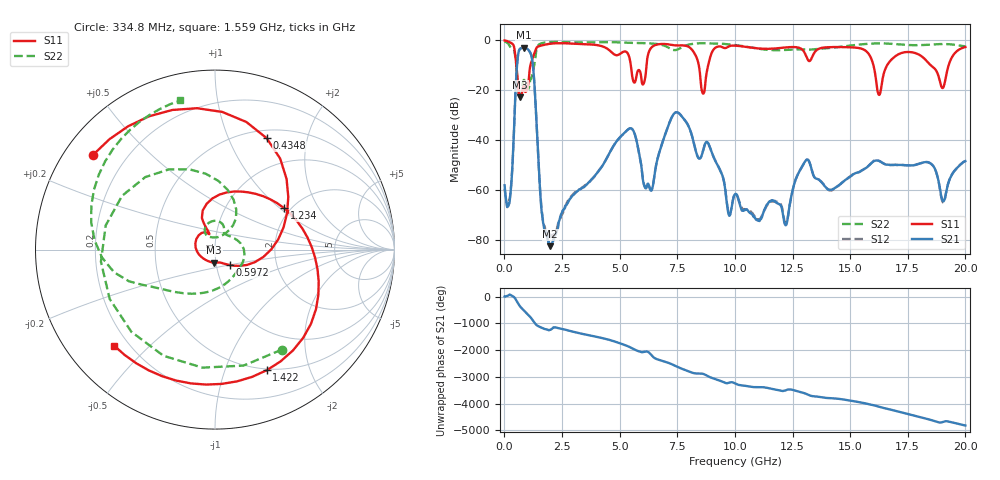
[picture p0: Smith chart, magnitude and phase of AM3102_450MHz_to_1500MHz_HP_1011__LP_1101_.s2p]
!Agilent Technologies,E8364B,MY43040894,A.07.50.67
!Agilent E8364B: A.07.50.67
!Date: Thursday, January 11, 2018 06:26:22
!Correction: S11(Full 2 Port(1,2))
!S21(Full 2 Port(1,2))
!S12(Full 2 Port(1,2))
!S22(Full 2 Port(1,2))
!S2P File: Measurements: S11, S21, S12, S22:
# Hz S  dB  R 50
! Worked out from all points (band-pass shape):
!   1601 points, 10 MHz to 20 GHz, reference 50 ohm
!   highest |S21| = -3.00 dB at 834.6 MHz (marker M1); lowest = -82.6 dB at 1.984 GHz (marker M2)
!   |S21| within 3 dB of the highest: 591.7 MHz to 1.167 GHz (575.5 MHz wide, 65.4 % of centre)
!   lowest |S11| = -22.8 dB at 684.7 MHz (marker M3), VSWR 1.16, Z = 49 - j7.14 ohm
!   |S11| at or under -10 dB: 521.4 MHz to 1.128 GHz (606.8 MHz wide, 73.6 % of centre); 5.485 GHz to 6.163 GHz (678.1 MHz wide, 11.6 % of centre); 18.5 GHz to 19.27 GHz (776.6 MHz wide, 4.11 % of centre)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
!   |S22| runs from -23.4 to -0.5 dB; largest |S21 - S12| = 0.00098
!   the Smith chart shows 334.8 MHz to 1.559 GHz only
!   S11 on the Smith chart (normalised r, x): 334.8 MHz: 0.08, +0.34; 434.8 MHz: 0.60, +1.39; 597.2 MHz: 1.16, -0.20; 1.234 GHz: 1.85, +1.07; 1.422 GHz: 0.49, -1.40; 1.559 GHz: 0.15, -0.39
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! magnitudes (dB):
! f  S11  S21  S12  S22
! 10 MHz  -0.1  -58.1  -59.5  -0.5
! 334.8 MHz  -1.3  -52.6  -52.6  -3.5
! 434.8 MHz  -3.3  -31.5  -31.5  -4.5
! 597.2 MHz  -18.5  -5.6  -5.6  -19.8
! 684.7 MHz  -22.8  -3.4  -3.4  -23.3
! 834.6 MHz  -18.3  -3.0  -3.0  -16.0
! 1.234 GHz  -6.9  -9.8  -9.8  -12.9
! 1.422 GHz  -2.7  -38.4  -38.4  -2.7
! 1.559 GHz  -2.2  -61.8  -61.5  -1.4
! 1.984 GHz  -1.4  -82.6  -77.9  -0.7
! 3.346 GHz  -1.5  -59.4  -59.2  -0.9
! 5.407 GHz  -6.4  -35.5  -35.5  -1.0
! 6.107 GHz  -15.1  -59.1  -59.0  -1.1
! 6.682 GHz  -1.6  -46.2  -46.2  -1.5
! 7.544 GHz  -2.0  -29.1  -29.1  -3.6
! 8.618 GHz  -21.4  -44.3  -44.3  -1.2
! 10.01 GHz  -2.1  -61.7  -61.8  -1.9
! 12.22 GHz  -2.8  -74.1  -73.0  -3.9
! 13.34 GHz  -6.9  -52.2  -52.3  -3.7
! 16.68 GHz  -9.0  -49.9  -50.0  -1.3
! 19.04 GHz  -18.9  -64.7  -65.0  -1.5
! 20 GHz  -2.7  -48.5  -48.4  -2.4
